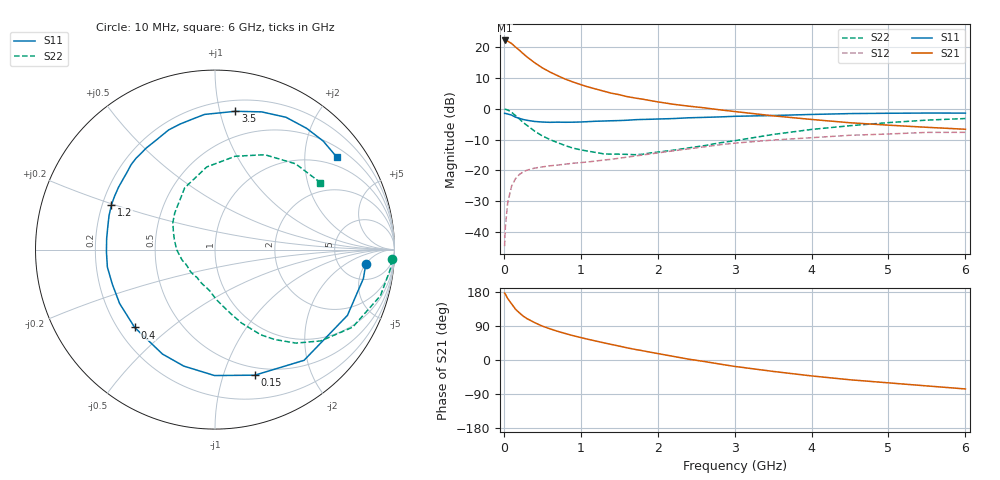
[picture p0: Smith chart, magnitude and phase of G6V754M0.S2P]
! SIEMENS Small Signal Semiconductors
! BFG193
! Si NPN RF Bipolar Junction Transistor in SOT223
! VCE = 0.75 V  IC = 4 mA
! Common Emitter S-Parameters:  August  1996
# GHz  S  MA  R  50
!  f  S11  S21  S12  S22
! GHz  MAG  ANG  MAG  ANG  MAG  ANG  MAG  ANG
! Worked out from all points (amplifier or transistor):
!   36 points, 10 MHz to 6 GHz, reference 50 ohm
!   highest |S21| = 22.2 dB at 10 MHz (marker M1)
!   |S21| within 3 dB of that: start of sweep to 194 MHz
!   unconditionally stable (mu >= 1): 1.125 GHz to 3.587 GHz
!   at 250 MHz: K = 0.30, MSG = 19.2 dB, |S12| = -20.5 dB
!   at 1.4 GHz: K = 1.11, MAG = 8.7 dB, |S12| = -16.4 dB
!   at 6 GHz: K = 1.00, MSG = 0.5 dB, |S12| = -7.6 dB
!   S11 on the Smith chart (normalised r, x): 10 MHz: 9, -5; 150 MHz: 0.42, -1.28; 400 MHz: 0.27, -0.38; 1.2 GHz: 0.24, +0.20; 3.5 GHz: 0.29, +1.12; 6 GHz: 0.74, +2.79
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0.01  0.8441 -5.4  12.87 176.4  0.0059 88.1  0.9865 -3.2
0.02  0.8424 -11.0  12.79 173.7  0.0122 84.1  0.9832 -6.3
0.05  0.8239 -26.4  12.51 162.3  0.0299 75.3  0.9567 -15.6
0.1  0.7916 -51.2  11.5 148.3  0.0551 64.6  0.8804 -29.4
0.15  0.734 -72.4  10.1 134.5  0.0731 53.7  0.7786 -40.8
0.2  0.7017 -90.2  8.98 124.8  0.0857 46.9  0.6891 -49.1
0.25  0.672 -105.0  7.88 116.1  0.0945 41.4  0.6016 -56.4
0.3  0.6514 -116.7  6.961 109.3  0.1009 37.7  0.5395 -61.7
0.4  0.6233 -135.9  5.601 98.7  0.1091 32.0  0.4344 -70.2
0.5  0.6105 -150.5  4.622 89.5  0.114 28.8  0.3633 -76.6
0.6  0.6037 -161.4  3.951 82.3  0.1189 27.2  0.3169 -82.2
0.7  0.6075 -170.8  3.444 75.7  0.1222 26.1  0.2823 -87.7
0.9  0.6068 174.1  2.723 64.3  0.1308 25.2  0.23 -97.7
1.1  0.6198 162.3  2.257 54.4  0.1377 25.2  0.2049 -109.8
1.2  0.6289 156.5  2.089 49.9  0.1424 25.3  0.1955 -115.9
1.6  0.6525 138.7  1.58 32.2  0.1643 24.2  0.1823 -141.9
2.2  0.6942 117.5  1.187 9.7  0.208 19.6  0.213 -179.7
2.8  0.7385 99.6  0.966 -10.5  0.2603 10.9  0.2795 147.2
3.5  0.7789 81.6  0.77 -30.1  0.3115 -4.0  0.3835 116.1
4.5  0.8367 61.8  0.594 -52.2  0.3722 -23.2  0.532 77.8
5.5  0.8539 45.1  0.501 -68.4  0.4143 -46.5  0.6557 46.8
6  0.852 37.3  0.466 -76.4  0.4148 -59.8  0.6956 32.5
